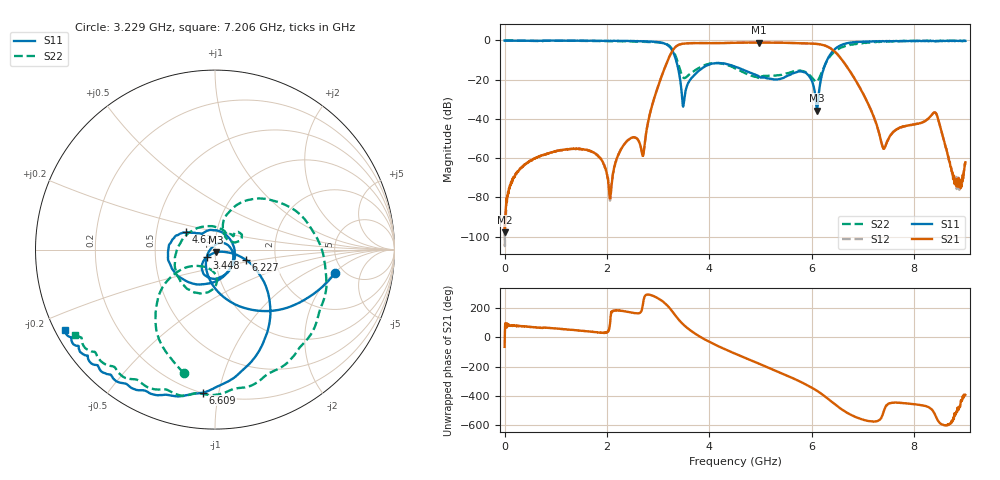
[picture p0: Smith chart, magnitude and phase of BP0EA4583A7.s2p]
!Agilent Technologies,E8358A,US40260310,A.06.04.32
!Agilent E8358A: A.06.04.32
!Date: Friday, November 22, 2019 00:21:13
!Correction: S11(Full 2 Port(1,2)) S21(Full 2 Port(1,2)) S12(Full 2 Port(1,2)) S22(Full 2 Port(1,2))
!S2P File: Measurements: S11, S21, S12, S22:
# Hz S  dB  R 50
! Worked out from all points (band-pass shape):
!   1601 points, 300 kHz to 9 GHz, reference 50 ohm
!   highest |S21| = -1.05 dB at 4.961 GHz (marker M1); lowest = -97.8 dB at 5.925 MHz (marker M2)
!   |S21| within 3 dB of the highest: 3.313 GHz to 6.37 GHz (3.056 GHz wide, 63.1 % of centre)
!   lowest |S11| = -35.7 dB at 6.103 GHz (marker M3), VSWR 1.03, Z = 50.4 - j1.59 ohm
!   |S11| at or under -10 dB: 3.348 GHz to 6.299 GHz (2.951 GHz wide, 61.2 % of centre)
!   |S22| runs from -21.1 to 0.0 dB; largest |S21 - S12| = 0.0099
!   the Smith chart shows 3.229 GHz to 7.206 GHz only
!   S11 on the Smith chart (normalised r, x): 3.229 GHz: 4.21, -2.03; 3.448 GHz: 0.91, -0.08; 4.63 GHz: 0.71, +0.14; 6.227 GHz: 1.40, -0.17; 6.609 GHz: 0.20, -0.90; 7.206 GHz: 0.03, -0.25
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300000  -0.06 -180.0  -92.39 -65.1  -90.93 -87.5  -0.01 -179.9
5924812  -0.07 179.9  -97.76 35.5  -104.83 127.9  -0.00 179.8
1.502125e9  -0.14 149.6  -55.55 44.9  -55.41 45.0  -0.22 120.5
2.070231e9  -0.16 132.1  -77.48 143.7  -80.35 144.3  -0.30 87.6
2.705835e9  -0.41 95.3  -58.75 -124.6  -58.68 -124.9  -0.65 18.1
3.00395e9  -0.94 55.7  -22.90 -94.9  -22.85 -94.6  -1.05 -38.4
3.228942e9  -3.36 -11.0  -7.68 -162.3  -7.66 -162.4  -2.99 -104.2
3.44831e9  -23.93 -136.7  -1.85 102.3  -1.79 102.2  -16.70 -141.6
3.847672e9  -14.37 -99.9  -1.34 -2.0  -1.29 -2.3  -13.32 -92.3
4.50015e9  -13.29 156.2  -1.17 -111.2  -1.13 -111.3  -14.20 168.0
4.629521e9  -14.60 148.9  -1.12 -130.4  -1.07 -130.6  -15.84 137.5
4.961385e9  -18.20 132.5  -1.05 -179.0  -1.01 -179.1  -19.09 56.7
5.523866e9  -18.04 -32.6  -1.24 97.3  -1.19 97.3  -16.68 40.0
6.001975e9  -20.58 -134.8  -1.62 15.8  -1.56 15.7  -18.95 20.8
6.103222e9  -35.71 -74.3  -1.80 -5.7  -1.76 -5.8  -20.91 50.1
6.226967e9  -14.82 -18.4  -2.36 -35.6  -2.32 -35.8  -14.10 72.1
6.609455e9  -1.94 -94.7  -10.51 -137.9  -10.53 -138.3  -3.30 -32.8
7.205685e9  -0.47 -151.6  -38.63 144.3  -38.54 144.6  -0.80 -148.5
7.5038e9  -0.34 -164.0  -49.82 -92.3  -49.78 -93.4  -0.57 -172.4
8.40377e9  -0.42 172.0  -36.69 -165.7  -36.64 -166.3  -0.30 160.5
8.791882e9  -0.35 164.9  -73.26 -174.7  -71.14 173.1  -0.14 154.6
9e9  -0.26 162.5  -62.07 -33.2  -62.68 -34.1  -0.22 150.5
